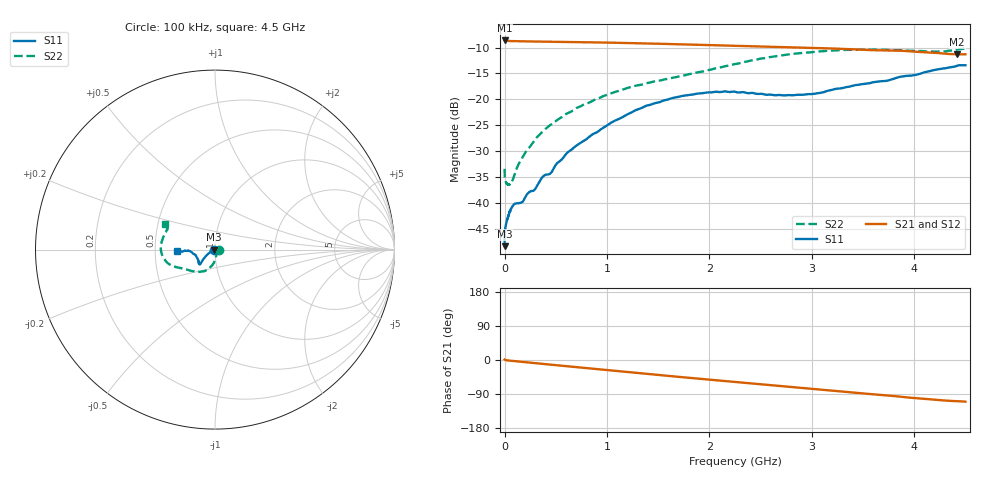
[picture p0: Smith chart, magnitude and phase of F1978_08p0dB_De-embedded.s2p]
! Integrated Device Technology
! Corporate Headquarters
! 6024 Silver Creek Valley Road
! San Jose, CA 95138  USA
! Phone:  1-408-284-8200
! Toll Free:  1-800-223-1366
! Webpage:  http://www.idt.com/
! Timing and RF Division
! 515 Groton Road, Suite 102
! Westford, MA 01886-6024
! Device:  F1978
! Description: 6-bit, 75 ohm, 0.5 dB Digital Step Attenuator
! Frequency:  5.0 MHz -  3.00 GHz
! Package:  4x4 mm QFN Plastic Package: 20 pin
! Ports:  2 RF, 11 DC
!  Pin  1  = D5 (16 dB)
!  Pin  2  = RF1  =  Port 1
!  Pin  3  = Serial Data In (DATA)
!  Pin  4  = Serial Clock (CLK)
!  Pin  5  = Serial Latch Enable (LE)
!  Pin  6  = VDD
!  Pin  7  = NC
!  Pin  8  = NC
!  Pin  9  = NC
!  Pin 10  = GND
!  Pin 11  = GND
!  Pin 12  = NC
!  Pin 13  = VMODE
!  Pin 14  = RF2  =  Port 2
!  Pin 15  = D4 (8 dB)
!  Pin 16  = D3 (4 dB)
!  Pin 17  = D2 (2 dB)
!  Pin 18  = NC
!  Pin 19  = D1 (1 dB)
!  Pin 20  = D0 (0.5 dB)
! State:  16
! Atten State:  8.0 dB
! Voltage:  +3.30 Volts
! Current:  0.591 mA
! Data:  The device was measured on a F1975 evaluation board which has
!  individual transmission lines to the RF pins.  Data was collected
!  using a calibrated network analyzer.  The evaluation board was
!  de-embedded using Automatic Fixture Removal (AFR).
!  The reference plane is the edge of the package pin.
! Misc:
!  Action Tracker AT0416
! Date Measured:  2018-02-08
! Date:  2018-03-26  MJV
! Note:
!  Integrated Device Technology supplies this data as a sample of measured
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# GHz S dB R 75
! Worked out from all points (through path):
!   291 points, 100 kHz to 4.5 GHz, reference 75 ohm
!   highest |S21| = -8.63 dB at 100 kHz (marker M1); lowest = -11.3 dB at 4.42 GHz (marker M2)
!   group delay of S21, straight-line fit = 69.3 ps
!   lowest |S11| = -48.3 dB at 100 kHz (marker M3), VSWR 1.01, Z = 74.4 - j0.0124 ohm
!   |S11| at or under -10 dB: start of sweep to end of sweep
!   |S22| runs from -36.4 to -10.1 dB; largest |S21 - S12| = 0.00022
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0.0001  -48.28 -178.8  -8.63 1.2  -8.64 1.2  -33.38 -0.7
0.0004  -46.90 -174.9  -8.66 1.1  -8.65 1.1  -34.08 -3.5
0.0008  -46.14 -172.1  -8.67 1.0  -8.67 1.0  -34.51 -3.6
0.002  -45.68 -174.1  -8.68 0.8  -8.68 0.8  -35.04 -4.7
0.012  -44.20 -170.3  -8.71 -0.5  -8.71 -0.5  -35.92 -14.8
0.056  -41.49 -165.8  -8.75 -1.8  -8.75 -1.8  -36.33 -40.7
0.08  -40.49 -159.7  -8.76 -2.5  -8.76 -2.5  -35.49 -54.0
0.14  -39.99 -152.0  -8.79 -4.1  -8.79 -4.1  -32.35 -67.4
0.32  -36.55 -157.5  -8.85 -8.9  -8.85 -8.9  -27.19 -83.4
0.38  -34.75 -153.4  -8.86 -10.5  -8.86 -10.5  -26.06 -85.5
0.44  -34.39 -152.4  -8.88 -12.0  -8.88 -12.0  -25.02 -87.2
0.6  -30.52 -153.8  -8.93 -16.2  -8.92 -16.2  -22.81 -94.4
0.76  -28.14 -148.8  -8.97 -20.3  -8.97 -20.3  -21.13 -99.9
1.06  -24.26 -144.3  -9.07 -28.2  -9.07 -28.2  -18.68 -109.6
1.52  -20.48 -138.1  -9.26 -39.9  -9.26 -39.9  -16.35 -125.7
1.88  -18.88 -135.7  -9.46 -48.9  -9.46 -48.9  -14.79 -140.0
2.26  -18.57 -138.6  -9.65 -58.2  -9.65 -58.2  -13.15 -152.1
2.64  -19.20 -150.1  -9.85 -67.4  -9.85 -67.4  -11.72 -160.5
3.02  -18.92 -164.9  -10.08 -76.6  -10.08 -76.6  -10.85 -169.2
3.76  -16.27 -177.3  -10.55 -93.9  -10.54 -93.9  -10.48 170.2
4.42  -13.51 -176.4  -11.32 -108.7  -11.32 -108.7  -10.38 153.9
4.5  -13.41 -178.4  -11.29 -110.0  -11.29 -110.0  -10.12 152.6
